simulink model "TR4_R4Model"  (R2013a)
settings: Solver=ode45  StartTime=0  StopTime=0.1  FixedStep=1e-4
PreLoadFcn:
  | warning('off','sm:sli:setup:compile:LocalSolverNotSupported')
InitFcn:
  |  SimParam.IC = SM2_InitCondConstrFnc(RawParam,IC);
model workspace (MAT data in the model file):
  handle : class17 (value not decoded)
  handle : class17 (value not decoded)
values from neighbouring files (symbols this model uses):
  RawParam = RobotParamGather(ParamLib)    [main_TR4.m]    (also in DeltaModelMain_v2.m; main_TimeSimulation.m; MGI.m = y)
libraries: SM2_BallJointPartsLib x8, SM2_ForeArmPartsLib x8, SM2_ArmPartsLib x4, SM2_MotorPartsLib x4, ElecDriverLib x1, SM2_FramePartsLib x1, SM2_ToolPartsLib x1

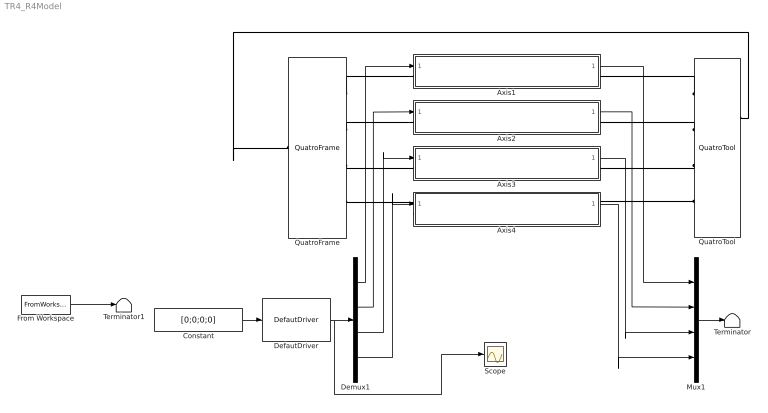
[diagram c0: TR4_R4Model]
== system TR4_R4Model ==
  Axis1 : Subsystem
  Axis2 : Subsystem
  Axis3 : Subsystem
  Axis4 : Subsystem
  Constant : Constant  Value=[0;0;0;0]
  DefautDriver : ElecDriverLib/DefautDriver  VariantControl=driverVarDefault
  Demux1 : Demux
  From Workspace : FromWorkspace  VariableName=simin  SampleTime=0
  Mux1 : Mux
  QuatroFrame : SM2_FramePartsLib/QuatroFrame
  QuatroTool : SM2_ToolPartsLib/QuatroTool
  Scope : Scope
  Terminator : Terminator
  Terminator1 : Terminator
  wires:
  Axis1/1(Alpha) -> Mux1/1
  Axis2/1(Alpha) -> Mux1/2
  Axis4/1(Alpha) -> Mux1/4
  Axis3/1(Alpha) -> Mux1/3
  Constant/1 -> DefautDriver/1
  From Workspace/1 -> Terminator1/1
  DefautDriver/1 -> Scope/1, Demux1/1
  Demux1/1 -> Axis1/1(Torque)
  Demux1/2 -> Axis2/1(Torque)
  Demux1/3 -> Axis3/1(Torque)
  Demux1/4 -> Axis4/1(Torque)
  Mux1/1 -> Terminator/1
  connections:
  QuatroFrame/RConn1 -- Axis1/LConn1
  QuatroFrame/RConn2 -- Axis2/LConn1
  QuatroFrame/RConn3 -- Axis3/LConn1
  QuatroTool/RConn3 -- Axis3/RConn1
  QuatroTool/RConn2 -- Axis2/RConn1
  QuatroTool/RConn1 -- Axis1/RConn1
  QuatroTool/LConn1 -- QuatroFrame/LConn1
  Axis4/LConn1 -- QuatroFrame/RConn4
  Axis4/RConn1 -- QuatroTool/RConn4

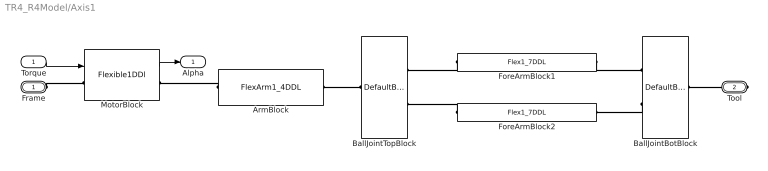
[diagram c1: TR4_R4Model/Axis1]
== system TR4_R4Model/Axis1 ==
  Torque : Inport
  ArmBlock : SM2_ArmPartsLib/FlexArm1_4DDL  VariantControl=armVarFlex1_4ddl
  BallJointBotBlock : SM2_BallJointPartsLib/DefaultBallJointBotPair
  BallJointTopBlock : SM2_BallJointPartsLib/DefaultBallJointTopPair
  ForeArmBlock1 : SM2_ForeArmPartsLib/Flex1_7DDL  VariantControl=foreArmVarFlex1_7ddl
  ForeArmBlock2 : SM2_ForeArmPartsLib/Flex1_7DDL  VariantControl=foreArmVarFlex1_7ddl
  MotorBlock : SM2_MotorPartsLib/Flexible1DDl  VariantControl=motorVarFlex1
      link override Revolute Joint: ClassName=RevoluteJoint  SenseConstraintForceX=off  SenseConstraintForceY=off  SenseConstraintForceZ=off  SenseConstraintTorqueX=off  SenseConstraintTorqueY=off  SenseConstraintTorqueZ=off  ConstraintWrenchDir=FollowerOnBase  ConstraintWrenchFrame=BaseFrame  EquilibriumPosition=SimParam.Motor.Alpha(AxisID)  EquilibriumPositionUnits=rad  SpringStiffness=SimParam.Motor.kSup  SpringStiffnessUnits=N*m/rad  DampingCoefficient=SimParam.Motor.c  DampingCoefficientUnits=N*m/(rad/s)  ActuationMode=TorqueForceActuation  SensePosition=on  SenseVelocity=off  SenseAcceleration=off  SenseTorqueForce=off  PositionTargetValue=SimParam.Motor.Alpha(AxisID)  PositionTargetValueUnits=rad  PositionTargetSpecify=on  PositionTargetPriority=High  VelocityTargetValue=0  VelocityTargetValueUnits=rad/s  VelocityTargetSpecify=on  VelocityTargetPriority=High  BlockFunction=simmechanics.library.joints.revolute_joint
  Frame : PMIOPort  Port=1  Side=Left
  Tool : PMIOPort  Port=2  Side=Right
  Alpha : Outport
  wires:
  Torque/1 -> MotorBlock/1
  MotorBlock/1 -> Alpha/1
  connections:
  ArmBlock/LConn1 -- MotorBlock/RConn1
  Frame/RConn1 -- MotorBlock/LConn1
  BallJointTopBlock/RConn1 -- ArmBlock/RConn1
  Tool/RConn1 -- BallJointBotBlock/RConn1
  ForeArmBlock2/LConn1 -- BallJointTopBlock/LConn2
  ForeArmBlock1/LConn1 -- BallJointTopBlock/LConn1
  ForeArmBlock1/RConn1 -- BallJointBotBlock/LConn1
  BallJointBotBlock/LConn2 -- ForeArmBlock2/RConn1

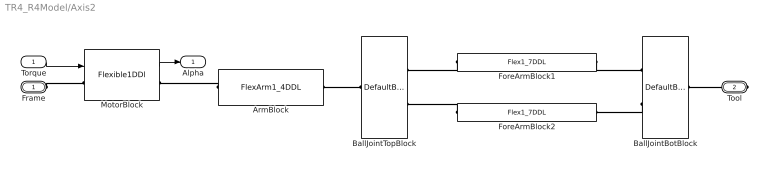
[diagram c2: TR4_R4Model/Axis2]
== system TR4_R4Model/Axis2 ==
  Torque : Inport
  ArmBlock : SM2_ArmPartsLib/FlexArm1_4DDL  VariantControl=armVarFlex1_4ddl
  BallJointBotBlock : SM2_BallJointPartsLib/DefaultBallJointBotPair
  BallJointTopBlock : SM2_BallJointPartsLib/DefaultBallJointTopPair
  ForeArmBlock1 : SM2_ForeArmPartsLib/Flex1_7DDL  VariantControl=foreArmVarFlex1_7ddl
  ForeArmBlock2 : SM2_ForeArmPartsLib/Flex1_7DDL  VariantControl=foreArmVarFlex1_7ddl
  MotorBlock : SM2_MotorPartsLib/Flexible1DDl  VariantControl=motorVarFlex1
  Frame : PMIOPort  Port=1  Side=Left
  Tool : PMIOPort  Port=2  Side=Right
  Alpha : Outport
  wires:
  Torque/1 -> MotorBlock/1
  MotorBlock/1 -> Alpha/1
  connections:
  ArmBlock/LConn1 -- MotorBlock/RConn1
  Frame/RConn1 -- MotorBlock/LConn1
  BallJointTopBlock/RConn1 -- ArmBlock/RConn1
  Tool/RConn1 -- BallJointBotBlock/RConn1
  ForeArmBlock2/LConn1 -- BallJointTopBlock/LConn2
  ForeArmBlock1/LConn1 -- BallJointTopBlock/LConn1
  ForeArmBlock1/RConn1 -- BallJointBotBlock/LConn1
  BallJointBotBlock/LConn2 -- ForeArmBlock2/RConn1

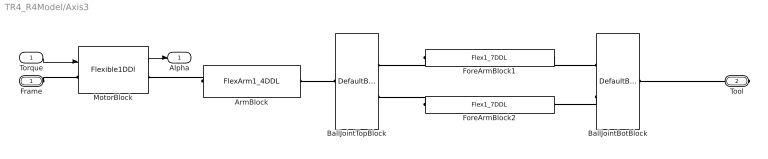
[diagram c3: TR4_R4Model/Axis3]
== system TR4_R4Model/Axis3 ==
  Torque : Inport
  ArmBlock : SM2_ArmPartsLib/FlexArm1_4DDL  VariantControl=armVarFlex1_4ddl
  BallJointBotBlock : SM2_BallJointPartsLib/DefaultBallJointBotPair
  BallJointTopBlock : SM2_BallJointPartsLib/DefaultBallJointTopPair
  ForeArmBlock1 : SM2_ForeArmPartsLib/Flex1_7DDL  VariantControl=foreArmVarFlex1_7ddl
  ForeArmBlock2 : SM2_ForeArmPartsLib/Flex1_7DDL  VariantControl=foreArmVarFlex1_7ddl
  MotorBlock : SM2_MotorPartsLib/Flexible1DDl  VariantControl=motorVarFlex1
  Frame : PMIOPort  Port=1  Side=Left
  Tool : PMIOPort  Port=2  Side=Right
  Alpha : Outport
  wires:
  Torque/1 -> MotorBlock/1
  MotorBlock/1 -> Alpha/1
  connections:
  ArmBlock/LConn1 -- MotorBlock/RConn1
  Frame/RConn1 -- MotorBlock/LConn1
  BallJointTopBlock/RConn1 -- ArmBlock/RConn1
  Tool/RConn1 -- BallJointBotBlock/RConn1
  ForeArmBlock2/LConn1 -- BallJointTopBlock/LConn2
  ForeArmBlock1/LConn1 -- BallJointTopBlock/LConn1
  ForeArmBlock1/RConn1 -- BallJointBotBlock/LConn1
  BallJointBotBlock/LConn2 -- ForeArmBlock2/RConn1

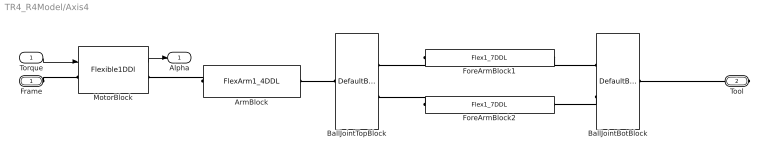
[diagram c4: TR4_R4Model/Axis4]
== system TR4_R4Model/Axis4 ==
  Torque : Inport
  ArmBlock : SM2_ArmPartsLib/FlexArm1_4DDL  VariantControl=armVarFlex1_4ddl
  BallJointBotBlock : SM2_BallJointPartsLib/DefaultBallJointBotPair
  BallJointTopBlock : SM2_BallJointPartsLib/DefaultBallJointTopPair
  ForeArmBlock1 : SM2_ForeArmPartsLib/Flex1_7DDL  VariantControl=foreArmVarFlex1_7ddl
  ForeArmBlock2 : SM2_ForeArmPartsLib/Flex1_7DDL  VariantControl=foreArmVarFlex1_7ddl
  MotorBlock : SM2_MotorPartsLib/Flexible1DDl  VariantControl=motorVarFlex1
  Frame : PMIOPort  Port=1  Side=Left
  Tool : PMIOPort  Port=2  Side=Right
  Alpha : Outport
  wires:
  Torque/1 -> MotorBlock/1
  MotorBlock/1 -> Alpha/1
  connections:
  ArmBlock/LConn1 -- MotorBlock/RConn1
  Frame/RConn1 -- MotorBlock/LConn1
  BallJointTopBlock/RConn1 -- ArmBlock/RConn1
  Tool/RConn1 -- BallJointBotBlock/RConn1
  ForeArmBlock2/LConn1 -- BallJointTopBlock/LConn2
  ForeArmBlock1/LConn1 -- BallJointTopBlock/LConn1
  ForeArmBlock1/RConn1 -- BallJointBotBlock/LConn1
  BallJointBotBlock/LConn2 -- ForeArmBlock2/RConn1
